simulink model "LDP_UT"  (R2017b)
settings: Solver=FixedStepDiscrete  StartTime=0.0  StopTime=10.0  FixedStep=0.01  RelTol=1e-3  EnableMultiTasking=on
undefined symbols (not defined in the file): ASWTYPE_FALSE, ASWTYPE_TRUE, CaCDP_ChrgTempNTCVoltTable_mV, CaCDP_ChrgTempTable_C, CaLDP_InletWtTempTable_C, CaLDP_InletWtVolt_mV, CaLDP_OutletWtTempTable_C, CaLDP_OutletWtVolt_mV, CcLDP_CC2SplyVolt_mV, CcLDP_CC2Uncon2ConTi_ms, CcLDP_CC2VoltThd_mV, CcLDP_DCChrgNegTempHiThrd_C, CcLDP_DCChrgNegTempMaxThrd_mV, CcLDP_DCChrgNegTempMinThrd_mV, CcLDP_DCChrgPosTempHiThrd_C, CcLDP_DCChrgPosTempMaxThrd_mV, CcLDP_DCChrgPosTempMinThrd_mV, CcLDP_DCSplyOnDebTi_ms, CcLDP_DCWakeVolt_V, CcLDP_IntWtTempHiThrd_C, CcLDP_IntWtTempMaxThrd_mV, CcLDP_IntWtTempMinThrd_mV, CcLDP_OutWtTempHiThrd_C, CcLDP_OutWtTempMaxThrd_mV, CcLDP_OutWtTempMinThrd_mV, Enum_CTCCtrCtlConnMode, Enum_LDPCC2St, Enum_LDPChrgGunState, Enum_ODPCCState, LDP_CONST2_NUMB, LDP_RUNTIME_MS
libraries: AIWAYS_Powertrain_BMS_lib x82
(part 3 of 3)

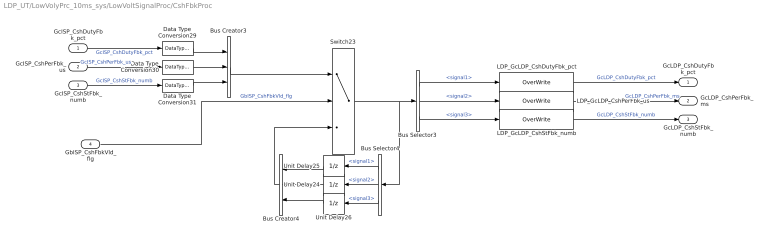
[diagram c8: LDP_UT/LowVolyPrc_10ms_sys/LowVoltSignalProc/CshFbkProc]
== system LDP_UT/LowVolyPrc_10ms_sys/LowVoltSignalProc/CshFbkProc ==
  GcISP_CshDutyFbk_pct : Inport
  GcISP_CshPerFbk_us : Inport  Port=2
  GcISP_CshStFbk_numb : Inport  Port=3
  GbISP_CshFbkVld_flg : Inport  Port=4
  Bus Creator3 : BusCreator  Inputs=3
  Bus Creator4 : BusCreator  Inputs=3
  Bus Selector3 : BusSelector  OutputSignals=signal1,signal2,signal3
  Bus Selector4 : BusSelector  OutputSignals=signal1,signal2,signal3
  Data Type Conversion29 : DataTypeConversion
  Data Type Conversion30 : DataTypeConversion
  Data Type Conversion31 : DataTypeConversion
  LDP_GcLDP_CshDutyFbk_pct : AIWAYS_Powertrain_BMS_lib/Signals/OverWrite  OverWrite_Value=CcLDP_CshDutyFbkOvr_pct  OverWrite_flag=CbLDP_CshDutyFbkOvrSwt_flg
  LDP_GcLDP_CshPerFbk_us : AIWAYS_Powertrain_BMS_lib/Signals/OverWrite  OverWrite_Value=CcLDP_CshPerFbkOvr_ms  OverWrite_flag=CbLDP_CshPerFbkOvrSwt_flg
  LDP_GcLDP_CshStFbk_numb : AIWAYS_Powertrain_BMS_lib/Signals/OverWrite  OverWrite_Value=CcLDP_CshStFbkOvr_numb  OverWrite_flag=CbLDP_CshStFbkOvrSwt_flg
  Switch23 : Switch  Criteria=u2 ~= 0  Threshold=1  RndMeth=Zero
  Unit Delay24 : UnitDelay  SampleTime=-1  StateName=StateName
  Unit Delay25 : UnitDelay  SampleTime=-1  StateName=StateName
  Unit Delay26 : UnitDelay  SampleTime=-1  StateName=StateName
  GcLDP_CshDutyFbk_pct : Outport
  GcLDP_CshPerFbk_ms : Outport  Port=2
  GcLDP_CshStFbk_numb : Outport  Port=3
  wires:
  Bus Selector4/2 -> Unit Delay24/1  "<signal2>"
  Bus Selector3/2 -> LDP_GcLDP_CshPerFbk_us/1  "<signal2>"
  LDP_GcLDP_CshDutyFbk_pct/1 -> GcLDP_CshDutyFbk_pct/1  "GcLDP_CshDutyFbk_pct"
  Bus Selector4/1 -> Unit Delay25/1  "<signal1>"
  Bus Selector3/1 -> LDP_GcLDP_CshDutyFbk_pct/1  "<signal1>"
  Unit Delay25/1 -> Bus Creator4/1
  Unit Delay26/1 -> Bus Creator4/3
  Unit Delay24/1 -> Bus Creator4/2
  GcISP_CshStFbk_numb/1 -> Data Type Conversion31/1  "GcISP_CshStFbk_numb"
  Bus Selector4/3 -> Unit Delay26/1  "<signal3>"
  GbISP_CshFbkVld_flg/1 -> Switch23/2  "GbISP_CshFbkVld_flg"
  Data Type Conversion31/1 -> Bus Creator3/3
  Data Type Conversion30/1 -> Bus Creator3/2
  Bus Creator3/1 -> Switch23/1
  Bus Selector3/3 -> LDP_GcLDP_CshStFbk_numb/1  "<signal3>"
  LDP_GcLDP_CshPerFbk_us/1 -> GcLDP_CshPerFbk_ms/1  "GcLDP_CshPerFbk_ms"
  Bus Creator4/1 -> Switch23/3
  GcISP_CshDutyFbk_pct/1 -> Data Type Conversion29/1  "GcISP_CshDutyFbk_pct"
  LDP_GcLDP_CshStFbk_numb/1 -> GcLDP_CshStFbk_numb/1  "GcLDP_CshStFbk_numb"
  Switch23/1 -> Bus Selector4/1, Bus Selector3/1
  GcISP_CshPerFbk_us/1 -> Data Type Conversion30/1  "GcISP_CshPerFbk_us"
  Data Type Conversion29/1 -> Bus Creator3/1

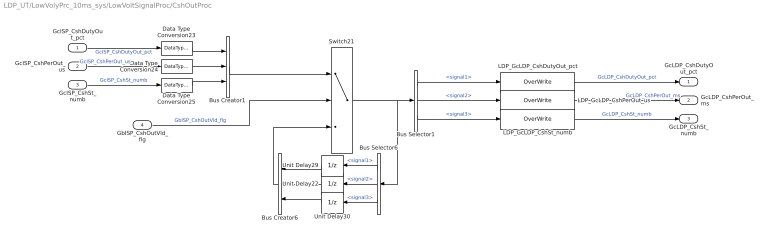
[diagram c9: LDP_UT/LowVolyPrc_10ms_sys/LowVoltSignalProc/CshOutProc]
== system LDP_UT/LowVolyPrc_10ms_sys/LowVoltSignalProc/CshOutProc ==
  GcISP_CshDutyOut_pct : Inport
  GcISP_CshPerOut_us : Inport  Port=2
  GcISP_CshSt_numb : Inport  Port=3
  GbISP_CshOutVld_flg : Inport  Port=4
  Bus Creator1 : BusCreator  Inputs=3
  Bus Creator6 : BusCreator  Inputs=3
  Bus Selector1 : BusSelector  OutputSignals=signal1,signal2,signal3
  Bus Selector6 : BusSelector  OutputSignals=signal1,signal2,signal3
  Data Type Conversion23 : DataTypeConversion
  Data Type Conversion24 : DataTypeConversion
  Data Type Conversion25 : DataTypeConversion
  LDP_GcLDP_CshDutyOut_pct : AIWAYS_Powertrain_BMS_lib/Signals/OverWrite  OverWrite_Value=CcLDP_CshDutyOutOvr_pct  OverWrite_flag=CbLDP_CshDutyOutOvrSwt_flg
  LDP_GcLDP_CshPerOut_us : AIWAYS_Powertrain_BMS_lib/Signals/OverWrite  OverWrite_Value=CcLDP_CshPerOutOvr_ms  OverWrite_flag=CbLDP_CshPerOutOvrSwt_flg
  LDP_GcLDP_CshSt_numb : AIWAYS_Powertrain_BMS_lib/Signals/OverWrite  OverWrite_Value=CcLDP_CshStOvr_numb  OverWrite_flag=CbLDP_CshStOvrSwt_flg
  Switch21 : Switch  Criteria=u2 ~= 0  Threshold=1  RndMeth=Zero
  Unit Delay22 : UnitDelay  SampleTime=-1  StateName=StateName
  Unit Delay29 : UnitDelay  SampleTime=-1  StateName=StateName
  Unit Delay30 : UnitDelay  SampleTime=-1  StateName=StateName
  GcLDP_CshDutyOut_pct : Outport
  GcLDP_CshPerOut_ms : Outport  Port=2
  GcLDP_CshSt_numb : Outport  Port=3
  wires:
  Data Type Conversion25/1 -> Bus Creator1/3
  Unit Delay22/1 -> Bus Creator6/2
  GcISP_CshSt_numb/1 -> Data Type Conversion25/1  "GcISP_CshSt_numb"
  Data Type Conversion23/1 -> Bus Creator1/1
  Bus Selector6/2 -> Unit Delay22/1  "<signal2>"
  Bus Creator6/1 -> Switch21/3
  Switch21/1 -> Bus Selector6/1, Bus Selector1/1
  LDP_GcLDP_CshDutyOut_pct/1 -> GcLDP_CshDutyOut_pct/1  "GcLDP_CshDutyOut_pct"
  Bus Selector6/1 -> Unit Delay29/1  "<signal1>"
  Unit Delay29/1 -> Bus Creator6/1
  Data Type Conversion24/1 -> Bus Creator1/2
  Bus Selector6/3 -> Unit Delay30/1  "<signal3>"
  Bus Selector1/2 -> LDP_GcLDP_CshPerOut_us/1  "<signal2>"
  GbISP_CshOutVld_flg/1 -> Switch21/2  "GbISP_CshOutVld_flg"
  Bus Selector1/1 -> LDP_GcLDP_CshDutyOut_pct/1  "<signal1>"
  Bus Selector1/3 -> LDP_GcLDP_CshSt_numb/1  "<signal3>"
  LDP_GcLDP_CshPerOut_us/1 -> GcLDP_CshPerOut_ms/1  "GcLDP_CshPerOut_ms"
  LDP_GcLDP_CshSt_numb/1 -> GcLDP_CshSt_numb/1  "GcLDP_CshSt_numb"
  Bus Creator1/1 -> Switch21/1
  GcISP_CshPerOut_us/1 -> Data Type Conversion24/1  "GcISP_CshPerOut_us"
  GcISP_CshDutyOut_pct/1 -> Data Type Conversion23/1  "GcISP_CshDutyOut_pct"
  Unit Delay30/1 -> Bus Creator6/3

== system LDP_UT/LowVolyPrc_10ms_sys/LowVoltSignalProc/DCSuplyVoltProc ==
  GcISP_DCSuplyVolt_mV : Inport
  GbISP_DCSuplyVoltVld_flg : Inport  Port=2
  Data Type Conversion1 : DataTypeConversion
  Data Type Conversion2 : DataTypeConversion
  Data Type Conversion4 : DataTypeConversion
  LDP_GbLDP_DCSuplyVoltVld_flg : AIWAYS_Powertrain_BMS_lib/Signals/OverWrite  OverWrite_Value=CbLDP_DCSuplyVoltVldOvr_flg  OverWrite_flag=CbLDP_DCSuplyVoltVldOvrSwt_flg
  LDP_GcLDP_DCSuplyVolt_mV : AIWAYS_Powertrain_BMS_lib/Signals/OverWrite  OverWrite_Value=CcLDP_DCSuplyVoltOvr_mV  OverWrite_flag=CbLDP_DCSuplyVoltOvrSwt_flg
  Switch4 : Switch  Criteria=u2 ~= 0
  Unit Delay4 : UnitDelay  SampleTime=-1  StateName=StateName
  GcLDP_DCSuplyVolt_mV : Outport
  GbLDP_DCSuplyVoltVld_flg : Outport  Port=2
  LbLDP_DCSuplyVoltVld_flg : Outport  Port=3
  LcLDP_DCSuplyVolt_mV : Outport  Port=4
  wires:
  Data Type Conversion4/1 -> Switch4/1
  Unit Delay4/1 -> Switch4/3
  Switch4/1 -> LDP_GcLDP_DCSuplyVolt_mV/1, Unit Delay4/1, Data Type Conversion2/1
  LDP_GcLDP_DCSuplyVolt_mV/1 -> GcLDP_DCSuplyVolt_mV/1  "GcLDP_DCSuplyVolt_mV"
  GbISP_DCSuplyVoltVld_flg/1 -> Data Type Conversion1/1, LDP_GbLDP_DCSuplyVoltVld_flg/1, Switch4/2  "GbISP_DCSuplyVoltVld_flg"
  GcISP_DCSuplyVolt_mV/1 -> Data Type Conversion4/1  "GcISP_DCSuplyVolt_mV"
  LDP_GbLDP_DCSuplyVoltVld_flg/1 -> GbLDP_DCSuplyVoltVld_flg/1  "GbLDP_DCSuplyVoltVld_flg"
  Data Type Conversion1/1 -> LbLDP_DCSuplyVoltVld_flg/1  "LbLDP_DCSuplyVoltVld_flg"
  Data Type Conversion2/1 -> LcLDP_DCSuplyVolt_mV/1  "LcLDP_DCSuplyVolt_mV"

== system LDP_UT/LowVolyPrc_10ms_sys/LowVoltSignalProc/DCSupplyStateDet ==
  LbLDP_DCSuplyVoltVld_flg : Inport
  LcLDP_DCSuplyVolt_mV : Inport  Port=2
  BMSDebounceStartZero1 : AIWAYS_Powertrain_BMS_lib/Debounce & Delay/BMSDebounceStartZero
  Constant1 : Constant  Value=ASWTYPE_TRUE
  KeMDPR_t_EngChrgBatIdleMinSetTm10 : Constant  Value=CcLDP_DCSplyOnDebTi_ms
  KeMDPR_t_EngChrgBatIdleMinSetTm2 : Constant  Value=LDP_RUNTIME_MS
  KeMDPR_t_EngChrgBatIdleMinSetTm3 : Constant  Value=LDP_RUNTIME_MS
  KeMDPR_t_EngChrgBatIdleMinSetTm6 : Constant  Value=CcLDP_DCWakeVolt_V
  KeMDPR_t_EngChrgBatIdleMinSetTm9 : Constant  Value=CcLDP_DCSplyOnDebTi_ms
  LDP_GbLDP_DC12VSply_flg : AIWAYS_Powertrain_BMS_lib/Signals/OverWrite  OverWrite_Value=CbLDP_DC12VSplyOvr_flg  OverWrite_flag=CbLDP_DC12VSplyOvrSwt_flg
  Logical Operator2 : Logic  AllPortsSameDT=off  OutDataTypeStr=boolean
  Relational Operator3 : RelationalOperator  OutDataTypeStr=boolean
  Relational Operator4 : RelationalOperator  Operator===  OutDataTypeStr=boolean
  GbLDP_DC12VSply_flg : Outport
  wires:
  LDP_GbLDP_DC12VSply_flg/1 -> GbLDP_DC12VSply_flg/1  "GbLDP_DC12VSply_flg"
  LcLDP_DCSuplyVolt_mV/1 -> Relational Operator3/1
  LbLDP_DCSuplyVoltVld_flg/1 -> Relational Operator4/1
  Constant1/1 -> Relational Operator4/2
  Relational Operator3/1 -> Logical Operator2/1
  Relational Operator4/1 -> Logical Operator2/2
  Logical Operator2/1 -> BMSDebounceStartZero1/1
  BMSDebounceStartZero1/1 -> LDP_GbLDP_DC12VSply_flg/1
  KeMDPR_t_EngChrgBatIdleMinSetTm2/1 -> BMSDebounceStartZero1/3
  KeMDPR_t_EngChrgBatIdleMinSetTm3/1 -> BMSDebounceStartZero1/5
  KeMDPR_t_EngChrgBatIdleMinSetTm6/1 -> Relational Operator3/2
  KeMDPR_t_EngChrgBatIdleMinSetTm9/1 -> BMSDebounceStartZero1/2
  KeMDPR_t_EngChrgBatIdleMinSetTm10/1 -> BMSDebounceStartZero1/4

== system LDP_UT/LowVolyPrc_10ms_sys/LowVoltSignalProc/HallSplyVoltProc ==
  GbISP_HallSplyVoltVld_flg : Inport
  GcISP_HallSplyVolt_mV : Inport  Port=2
  Data Type Conversion2 : DataTypeConversion
  LDP_GbLDP_HallSplyVoltVld_flg : AIWAYS_Powertrain_BMS_lib/Signals/OverWrite  OverWrite_Value=CbLDP_HallSplyVoltVldOvr_flg  OverWrite_flag=CbLDP_HallSplyVoltVldOvrSwt_flg
  LDP_GcLDP_HallSplyVolt_mV : AIWAYS_Powertrain_BMS_lib/Signals/OverWrite  OverWrite_Value=CcLDP_HallSplyVoltOvr_mV  OverWrite_flag=CbLDP_HallSplyVoltOvrSwt_flg
  Switch2 : Switch  Criteria=u2 ~= 0
  Unit Delay2 : UnitDelay  SampleTime=-1  StateName=StateName
  GcLDP_HallSplyVolt_mV : Outport
  GbLDP_HallSplyVoltVld_flg : Outport  Port=2
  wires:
  Data Type Conversion2/1 -> Switch2/1
  Unit Delay2/1 -> Switch2/3
  GbISP_HallSplyVoltVld_flg/1 -> LDP_GbLDP_HallSplyVoltVld_flg/1, Switch2/2  "GbISP_HallSplyVoltVld_flg"
  LDP_GbLDP_HallSplyVoltVld_flg/1 -> GbLDP_HallSplyVoltVld_flg/1  "GbLDP_HallSplyVoltVld_flg"
  GcISP_HallSplyVolt_mV/1 -> Data Type Conversion2/1  "GcISP_HallSplyVolt_mV"
  Switch2/1 -> Unit Delay2/1, LDP_GcLDP_HallSplyVolt_mV/1
  LDP_GcLDP_HallSplyVolt_mV/1 -> GcLDP_HallSplyVolt_mV/1  "GcLDP_HallSplyVolt_mV"

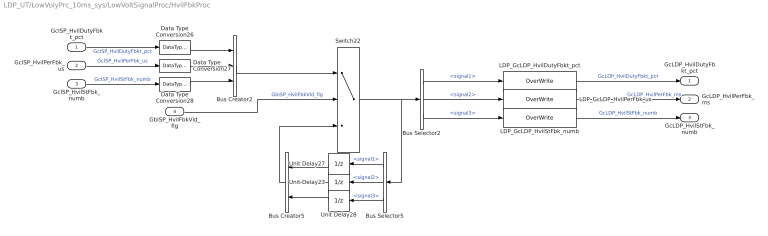
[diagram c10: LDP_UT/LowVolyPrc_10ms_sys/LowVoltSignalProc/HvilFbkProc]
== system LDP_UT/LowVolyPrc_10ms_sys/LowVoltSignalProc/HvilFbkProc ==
  GcISP_HvilDutyFbkt_pct : Inport
  GcISP_HvilPerFbk_us : Inport  Port=2
  GcISP_HvilStFbk_numb : Inport  Port=3
  GbISP_HvilFbkVld_flg : Inport  Port=4
  Bus Creator2 : BusCreator  Inputs=3
  Bus Creator5 : BusCreator  Inputs=3
  Bus Selector2 : BusSelector  OutputSignals=signal1,signal2,signal3
  Bus Selector5 : BusSelector  OutputSignals=signal1,signal2,signal3
  Data Type Conversion26 : DataTypeConversion
  Data Type Conversion27 : DataTypeConversion
  Data Type Conversion28 : DataTypeConversion
  LDP_GcLDP_HvilDutyFbkt_pct : AIWAYS_Powertrain_BMS_lib/Signals/OverWrite  OverWrite_Value=CcLDP_HvilDutyFbktOvr_pct  OverWrite_flag=CbLDP_HvilDutyFbktOvrSwt_flg
  LDP_GcLDP_HvilPerFbk_us : AIWAYS_Powertrain_BMS_lib/Signals/OverWrite  OverWrite_Value=CcLDP_HvilPerFbkOvr_ms  OverWrite_flag=CbLDP_HvilPerFbkOvrSwt_flg
  LDP_GcLDP_HvilStFbk_numb : AIWAYS_Powertrain_BMS_lib/Signals/OverWrite  OverWrite_Value=CcLDP_HvilStFbkOvr_numb  OverWrite_flag=CbLDP_HvilStFbkOvrSwt_flg
  Switch22 : Switch  Criteria=u2 ~= 0  Threshold=1  RndMeth=Zero
  Unit Delay23 : UnitDelay  SampleTime=-1  StateName=StateName
  Unit Delay27 : UnitDelay  SampleTime=-1  StateName=StateName
  Unit Delay28 : UnitDelay  SampleTime=-1  StateName=StateName
  GcLDP_HvilDutyFbkt_pct : Outport
  GcLDP_HvilPerFbk_ms : Outport  Port=2
  GcLDP_HvilStFbk_numb : Outport  Port=3
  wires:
  Switch22/1 -> Bus Selector5/1, Bus Selector2/1
  Data Type Conversion26/1 -> Bus Creator2/1
  Unit Delay23/1 -> Bus Creator5/2
  LDP_GcLDP_HvilStFbk_numb/1 -> GcLDP_HvilStFbk_numb/1  "GcLDP_HvilStFbk_numb"
  Bus Selector5/3 -> Unit Delay28/1  "<signal3>"
  Bus Selector5/2 -> Unit Delay23/1  "<signal2>"
  Bus Selector5/1 -> Unit Delay27/1  "<signal1>"
  Bus Creator5/1 -> Switch22/3
  Bus Selector2/2 -> LDP_GcLDP_HvilPerFbk_us/1  "<signal2>"
  Unit Delay28/1 -> Bus Creator5/3
  Unit Delay27/1 -> Bus Creator5/1
  GcISP_HvilDutyFbkt_pct/1 -> Data Type Conversion26/1  "GcISP_HvilDutyFbkt_pct"
  Data Type Conversion28/1 -> Bus Creator2/3
  Bus Creator2/1 -> Switch22/1
  Data Type Conversion27/1 -> Bus Creator2/2
  GcISP_HvilPerFbk_us/1 -> Data Type Conversion27/1  "GcISP_HvilPerFbk_us"
  LDP_GcLDP_HvilPerFbk_us/1 -> GcLDP_HvilPerFbk_ms/1  "GcLDP_HvilPerFbk_ms"
  LDP_GcLDP_HvilDutyFbkt_pct/1 -> GcLDP_HvilDutyFbkt_pct/1  "GcLDP_HvilDutyFbkt_pct"
  Bus Selector2/3 -> LDP_GcLDP_HvilStFbk_numb/1  "<signal3>"
  GcISP_HvilStFbk_numb/1 -> Data Type Conversion28/1  "GcISP_HvilStFbk_numb"
  Bus Selector2/1 -> LDP_GcLDP_HvilDutyFbkt_pct/1  "<signal1>"
  GbISP_HvilFbkVld_flg/1 -> Switch22/2  "GbISP_HvilFbkVld_flg"

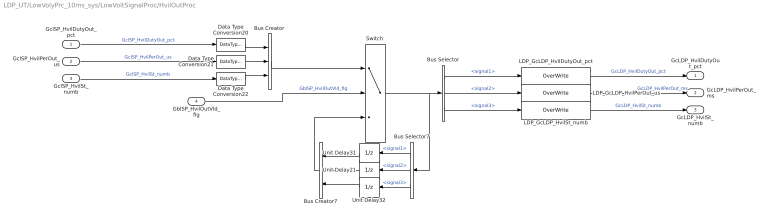
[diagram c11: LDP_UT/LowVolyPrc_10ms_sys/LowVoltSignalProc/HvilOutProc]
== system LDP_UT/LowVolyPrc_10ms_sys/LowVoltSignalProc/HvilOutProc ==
  GcISP_HvilDutyOut_pct : Inport
  GcISP_HvilPerOut_us : Inport  Port=2
  GcISP_HvilSt_numb : Inport  Port=3
  GbISP_HvilOutVld_flg : Inport  Port=4
  Bus Creator : BusCreator  Inputs=3
  Bus Creator7 : BusCreator  Inputs=3
  Bus Selector : BusSelector  OutputSignals=signal1,signal2,signal3
  Bus Selector7 : BusSelector  OutputSignals=signal1,signal2,signal3
  Data Type Conversion20 : DataTypeConversion
  Data Type Conversion21 : DataTypeConversion
  Data Type Conversion22 : DataTypeConversion
  LDP_GcLDP_HvilDutyOut_pct : AIWAYS_Powertrain_BMS_lib/Signals/OverWrite  OverWrite_Value=CcLDP_HvilDutyOutOvr_pct  OverWrite_flag=CbLDP_HvilDutyOutOvrSwt_flg
  LDP_GcLDP_HvilPerOut_us : AIWAYS_Powertrain_BMS_lib/Signals/OverWrite  OverWrite_Value=CcLDP_HvilPerOutOvr_ms  OverWrite_flag=CbLDP_HvilPerOutOvrSwt_flg
  LDP_GcLDP_HvilSt_numb : AIWAYS_Powertrain_BMS_lib/Signals/OverWrite  OverWrite_Value=CcLDP_HvilStOvr_numb  OverWrite_flag=CbLDP_HvilStOvrSwt_flg
  Switch : Switch  Criteria=u2 ~= 0  Threshold=1  RndMeth=Zero
  Unit Delay21 : UnitDelay  SampleTime=-1  StateName=StateName
  Unit Delay31 : UnitDelay  SampleTime=-1  StateName=StateName
  Unit Delay32 : UnitDelay  SampleTime=-1  StateName=StateName
  GcLDP_HvilDutyOut_pct : Outport
  GcLDP_HvilPerOut_ms : Outport  Port=2
  GcLDP_HvilSt_numb : Outport  Port=3
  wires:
  Bus Selector/1 -> LDP_GcLDP_HvilDutyOut_pct/1  "<signal1>"
  Bus Selector7/2 -> Unit Delay21/1  "<signal2>"
  Unit Delay32/1 -> Bus Creator7/3
  Bus Selector7/1 -> Unit Delay31/1  "<signal1>"
  Bus Creator7/1 -> Switch/3
  GcISP_HvilDutyOut_pct/1 -> Data Type Conversion20/1  "GcISP_HvilDutyOut_pct"
  Unit Delay21/1 -> Bus Creator7/2
  Unit Delay31/1 -> Bus Creator7/1
  GbISP_HvilOutVld_flg/1 -> Switch/2  "GbISP_HvilOutVld_flg"
  GcISP_HvilSt_numb/1 -> Data Type Conversion22/1  "GcISP_HvilSt_numb"
  Data Type Conversion22/1 -> Bus Creator/3
  Switch/1 -> Bus Selector7/1, Bus Selector/1
  Bus Selector/3 -> LDP_GcLDP_HvilSt_numb/1  "<signal3>"
  Bus Creator/1 -> Switch/1
  LDP_GcLDP_HvilPerOut_us/1 -> GcLDP_HvilPerOut_ms/1  "GcLDP_HvilPerOut_ms"
  Bus Selector7/3 -> Unit Delay32/1  "<signal3>"
  Data Type Conversion20/1 -> Bus Creator/1
  Bus Selector/2 -> LDP_GcLDP_HvilPerOut_us/1  "<signal2>"
  LDP_GcLDP_HvilSt_numb/1 -> GcLDP_HvilSt_numb/1  "GcLDP_HvilSt_numb"
  LDP_GcLDP_HvilDutyOut_pct/1 -> GcLDP_HvilDutyOut_pct/1  "GcLDP_HvilDutyOut_pct"
  GcISP_HvilPerOut_us/1 -> Data Type Conversion21/1  "GcISP_HvilPerOut_us"
  Data Type Conversion21/1 -> Bus Creator/2

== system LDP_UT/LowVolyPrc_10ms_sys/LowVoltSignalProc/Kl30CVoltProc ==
  GcISP_Kl30CVolt_mV : Inport
  GbISP_Kl30CVoltVld_flg : Inport  Port=2
  Data Type Conversion5 : DataTypeConversion
  LDP_GbLDP_Kl30CVoltVld_flg : AIWAYS_Powertrain_BMS_lib/Signals/OverWrite  OverWrite_Value=CbLDP_Kl30CVoltVldOvr_flg  OverWrite_flag=CbLDP_Kl30CVoltVldOvrSwt_flg
  LDP_GcLDP_Kl30CVolt_mV : AIWAYS_Powertrain_BMS_lib/Signals/OverWrite  OverWrite_Value=CcLDP_Kl30CVoltOvr_mV  OverWrite_flag=CbLDP_Kl30CVoltOvrSwt_flg
  Switch5 : Switch  Criteria=u2 ~= 0
  Unit Delay5 : UnitDelay  SampleTime=-1  StateName=StateName
  GcLDP_Kl30CVolt_mV : Outport
  GbLDP_Kl30CVoltVld_flg : Outport  Port=2
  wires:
  GcISP_Kl30CVolt_mV/1 -> Data Type Conversion5/1  "GcISP_Kl30CVolt_mV"
  Switch5/1 -> LDP_GcLDP_Kl30CVolt_mV/1, Unit Delay5/1
  Unit Delay5/1 -> Switch5/3
  GbISP_Kl30CVoltVld_flg/1 -> Switch5/2, LDP_GbLDP_Kl30CVoltVld_flg/1  "GbISP_Kl30CVoltVld_flg"
  LDP_GcLDP_Kl30CVolt_mV/1 -> GcLDP_Kl30CVolt_mV/1  "GcLDP_Kl30CVolt_mV"
  LDP_GbLDP_Kl30CVoltVld_flg/1 -> GbLDP_Kl30CVoltVld_flg/1  "GbLDP_Kl30CVoltVld_flg"
  Data Type Conversion5/1 -> Switch5/1

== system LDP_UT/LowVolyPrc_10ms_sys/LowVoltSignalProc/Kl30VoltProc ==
  GbISP_Kl30VoltVld_flg : Inport
  GcISP_Kl30Volt_mV : Inport  Port=2
  Data Type Conversion6 : DataTypeConversion
  LDP_GbLDP_Kl30VoltVld_flg : AIWAYS_Powertrain_BMS_lib/Signals/OverWrite  OverWrite_Value=CbLDP_Kl30VoltVldOvr_flg  OverWrite_flag=CbLDP_Kl30VoltVldOvrSwt_flg
  LDP_GcLDP_Kl30Volt_mV : AIWAYS_Powertrain_BMS_lib/Signals/OverWrite  OverWrite_Value=CcLDP_Kl30VoltOvr_mV  OverWrite_flag=CbLDP_Kl30VoltOvrSwt_flg
  Switch6 : Switch  Criteria=u2 ~= 0
  Unit Delay6 : UnitDelay  SampleTime=-1  StateName=StateName
  GcLDP_Kl30Volt_mV : Outport
  GbLDP_Kl30VoltVld_flg : Outport  Port=2
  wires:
  LDP_GbLDP_Kl30VoltVld_flg/1 -> GbLDP_Kl30VoltVld_flg/1  "GbLDP_Kl30VoltVld_flg"
  GbISP_Kl30VoltVld_flg/1 -> LDP_GbLDP_Kl30VoltVld_flg/1, Switch6/2  "GbISP_Kl30VoltVld_flg"
  Unit Delay6/1 -> Switch6/3
  LDP_GcLDP_Kl30Volt_mV/1 -> GcLDP_Kl30Volt_mV/1  "GcLDP_Kl30Volt_mV"
  GcISP_Kl30Volt_mV/1 -> Data Type Conversion6/1  "GcISP_Kl30Volt_mV"
  Switch6/1 -> LDP_GcLDP_Kl30Volt_mV/1, Unit Delay6/1
  Data Type Conversion6/1 -> Switch6/1

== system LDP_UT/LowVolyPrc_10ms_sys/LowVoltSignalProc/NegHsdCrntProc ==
  GcISP_NegHsdCrnt_mV : Inport
  GbISP_NegHsdCrntVld_flg : Inport  Port=2
  Data Type Conversion9 : DataTypeConversion
  LDP_GbLDP_NegHsdCrntVld_flg : AIWAYS_Powertrain_BMS_lib/Signals/OverWrite  OverWrite_Value=CbLDP_NegHsdCrntVldOvr_flg  OverWrite_flag=CbLDP_NegHsdCrntVldOvrSwt_flg
  LDP_GcLDP_NegHsdCrnt_mV : AIWAYS_Powertrain_BMS_lib/Signals/OverWrite  OverWrite_Value=CcLDP_NegHsdCrntOvr_mV  OverWrite_flag=CbLDP_NegHsdCrntOvrSwt_flg
  Switch9 : Switch  Criteria=u2 ~= 0
  Unit Delay9 : UnitDelay  SampleTime=-1  StateName=StateName
  GcLDP_NegHsdCrnt_mV : Outport
  GbLDP_NegHsdCrntVld_flg : Outport  Port=2
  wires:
  Switch9/1 -> LDP_GcLDP_NegHsdCrnt_mV/1, Unit Delay9/1
  LDP_GbLDP_NegHsdCrntVld_flg/1 -> GbLDP_NegHsdCrntVld_flg/1  "GbLDP_NegHsdCrntVld_flg"
  Unit Delay9/1 -> Switch9/3
  LDP_GcLDP_NegHsdCrnt_mV/1 -> GcLDP_NegHsdCrnt_mV/1  "GcLDP_NegHsdCrnt_mV"
  GcISP_NegHsdCrnt_mV/1 -> Data Type Conversion9/1  "GcISP_NegHsdCrnt_mV"
  GbISP_NegHsdCrntVld_flg/1 -> LDP_GbLDP_NegHsdCrntVld_flg/1, Switch9/2  "GbISP_NegHsdCrntVld_flg"
  Data Type Conversion9/1 -> Switch9/1

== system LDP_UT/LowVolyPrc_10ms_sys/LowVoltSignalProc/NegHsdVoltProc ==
  GcISP_NegHsdVolt_mV : Inport
  GbISP_NegHsdVoltVld_flg : Inport  Port=2
  Data Type Conversion11 : DataTypeConversion
  LDP_GbLDP_NegHsdVoltVld_flg : AIWAYS_Powertrain_BMS_lib/Signals/OverWrite  OverWrite_Value=CbLDP_NegHsdVoltVldOvr_flg  OverWrite_flag=CbLDP_NegHsdVoltVldOvrSwt_flg
  LDP_GcLDP_NegHsdVolt_mV : AIWAYS_Powertrain_BMS_lib/Signals/OverWrite  OverWrite_Value=CcLDP_NegHsdVoltOvr_mV  OverWrite_flag=CbLDP_NegHsdVoltOvrSwt_flg
  Switch11 : Switch  Criteria=u2 ~= 0
  Unit Delay11 : UnitDelay  SampleTime=-1  StateName=StateName
  GcLDP_NegHsdVolt_mV : Outport
  GbLDP_NegHsdVoltVld_flg : Outport  Port=2
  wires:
  LDP_GbLDP_NegHsdVoltVld_flg/1 -> GbLDP_NegHsdVoltVld_flg/1  "GbLDP_NegHsdVoltVld_flg"
  Unit Delay11/1 -> Switch11/3
  Data Type Conversion11/1 -> Switch11/1
  GbISP_NegHsdVoltVld_flg/1 -> LDP_GbLDP_NegHsdVoltVld_flg/1, Switch11/2  "GbISP_NegHsdVoltVld_flg"
  Switch11/1 -> LDP_GcLDP_NegHsdVolt_mV/1, Unit Delay11/1
  LDP_GcLDP_NegHsdVolt_mV/1 -> GcLDP_NegHsdVolt_mV/1  "GcLDP_NegHsdVolt_mV"
  GcISP_NegHsdVolt_mV/1 -> Data Type Conversion11/1  "GcISP_NegHsdVolt_mV"

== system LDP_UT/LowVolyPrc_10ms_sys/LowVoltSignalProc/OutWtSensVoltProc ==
  GcISP_OutWtSensVolt_mV : Inport
  GbISP_OutWtSensVoltVld_flg : Inport  Port=2
  1-D Lookup Table3 : Lookup_n-D  NumberOfTableDimensions=1  BreakpointsForDimension1=CaLDP_OutletWtVolt_mV  Table=CaLDP_OutletWtTempTable_C  ExtrapMethod=Clip  UseLastTableValue=on  InternalRulePriority=Speed  OutDataTypeStr=Inherit: Inherit from 'Table data'  RndMeth=Simplest
  Data Type Conversion17 : DataTypeConversion
  LDP_GbLDP_OutWtSensVoltVld_flg : AIWAYS_Powertrain_BMS_lib/Signals/OverWrite  OverWrite_Value=CbLDP_OutWtSensVoltVldOvr_flg  OverWrite_flag=CbLDP_OutWtSensVoltVldOvrSwt_flg
  LDP_GcLDP_OutWtTemp_C : AIWAYS_Powertrain_BMS_lib/Signals/OverWrite  OverWrite_Value=CcLDP_OutWtTempOvr_C  OverWrite_flag=CbLDP_OutWtTempOvrSwt_flg
  Switch17 : Switch  Criteria=u2 ~= 0
  Unit Delay17 : UnitDelay  SampleTime=-1  StateName=StateName
  GbLDP_OutWtSensVoltVld_flg : Outport
  GcLDP_OutWtTemp_C : Outport  Port=2
  LcLDP_OutWtSensVolt_mV : Outport  Port=3
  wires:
  Data Type Conversion17/1 -> Switch17/1
  GbISP_OutWtSensVoltVld_flg/1 -> LDP_GbLDP_OutWtSensVoltVld_flg/1, Switch17/2  "GbISP_OutWtSensVoltVld_flg"
  LDP_GbLDP_OutWtSensVoltVld_flg/1 -> GbLDP_OutWtSensVoltVld_flg/1  "GbLDP_OutWtSensVoltVld_flg"
  Unit Delay17/1 -> Switch17/3
  GcISP_OutWtSensVolt_mV/1 -> Data Type Conversion17/1  "GcISP_OutWtSensVolt_mV"
  Switch17/1 -> 1-D Lookup Table3/1, LcLDP_OutWtSensVolt_mV/1, Unit Delay17/1  "LcLDP_OutWtSensVolt_mV"
  LDP_GcLDP_OutWtTemp_C/1 -> GcLDP_OutWtTemp_C/1  "GcLDP_OutWtTemp_C"
  1-D Lookup Table3/1 -> LDP_GcLDP_OutWtTemp_C/1

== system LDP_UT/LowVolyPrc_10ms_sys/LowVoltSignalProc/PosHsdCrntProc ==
  GcISP_PosHsdCrnt_mV : Inport
  GbISP_PosHsdCrntVld_flg : Inport  Port=2
  Data Type Conversion7 : DataTypeConversion
  LDP_GbLDP_PosHsdCrntVld_flg : AIWAYS_Powertrain_BMS_lib/Signals/OverWrite  OverWrite_Value=CbLDP_PosHsdCrntVldOvr_flg  OverWrite_flag=CbLDP_PosHsdCrntVldOvrSwt_flg
  LDP_GcLDP_PosHsdCrnt_mV : AIWAYS_Powertrain_BMS_lib/Signals/OverWrite  OverWrite_Value=CcLDP_PosHsdCrntOvr_mV  OverWrite_flag=CbLDP_PosHsdCrntOvrSwt_flg
  Switch7 : Switch  Criteria=u2 ~= 0
  Unit Delay7 : UnitDelay  SampleTime=-1  StateName=StateName
  GcLDP_PosHsdCrnt_mV : Outport
  GbLDP_PosHsdCrntVld_flg : Outport  Port=2
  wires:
  Switch7/1 -> LDP_GcLDP_PosHsdCrnt_mV/1, Unit Delay7/1
  GbISP_PosHsdCrntVld_flg/1 -> LDP_GbLDP_PosHsdCrntVld_flg/1, Switch7/2  "GbISP_PosHsdCrntVld_flg"
  GcISP_PosHsdCrnt_mV/1 -> Data Type Conversion7/1  "GcISP_PosHsdCrnt_mV"
  LDP_GbLDP_PosHsdCrntVld_flg/1 -> GbLDP_PosHsdCrntVld_flg/1  "GbLDP_PosHsdCrntVld_flg"
  LDP_GcLDP_PosHsdCrnt_mV/1 -> GcLDP_PosHsdCrnt_mV/1  "GcLDP_PosHsdCrnt_mV"
  Data Type Conversion7/1 -> Switch7/1
  Unit Delay7/1 -> Switch7/3

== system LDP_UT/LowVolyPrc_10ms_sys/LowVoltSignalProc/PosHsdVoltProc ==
  GcISP_PosHsdVolt_mV : Inport
  GbISP_PosHsdVoltVld_flg : Inport  Port=2
  Data Type Conversion10 : DataTypeConversion
  LDP_GbLDP_PosHsdVoltVld_flg : AIWAYS_Powertrain_BMS_lib/Signals/OverWrite  OverWrite_Value=CbLDP_PosHsdVoltVldOvr_flg  OverWrite_flag=CbLDP_PosHsdVoltVldOvrSwt_flg
  LDP_GcLDP_PosHsdVolt_mV : AIWAYS_Powertrain_BMS_lib/Signals/OverWrite  OverWrite_Value=CcLDP_PosHsdVoltOvr_mV  OverWrite_flag=CbLDP_PosHsdVoltOvrSwt_flg
  Switch10 : Switch  Criteria=u2 ~= 0
  Unit Delay10 : UnitDelay  SampleTime=-1  StateName=StateName
  GcLDP_PosHsdVolt_mV : Outport
  GbLDP_PosHsdVoltVld_flg : Outport  Port=2
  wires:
  LDP_GbLDP_PosHsdVoltVld_flg/1 -> GbLDP_PosHsdVoltVld_flg/1  "GbLDP_PosHsdVoltVld_flg"
  GcISP_PosHsdVolt_mV/1 -> Data Type Conversion10/1  "GcISP_PosHsdVolt_mV"
  Data Type Conversion10/1 -> Switch10/1
  Unit Delay10/1 -> Switch10/3
  GbISP_PosHsdVoltVld_flg/1 -> LDP_GbLDP_PosHsdVoltVld_flg/1, Switch10/2  "GbISP_PosHsdVoltVld_flg"
  LDP_GcLDP_PosHsdVolt_mV/1 -> GcLDP_PosHsdVolt_mV/1  "GcLDP_PosHsdVolt_mV"
  Switch10/1 -> LDP_GcLDP_PosHsdVolt_mV/1, Unit Delay10/1

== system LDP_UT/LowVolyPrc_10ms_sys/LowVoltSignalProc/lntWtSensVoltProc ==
  GcISP_lntWtSensVolt_mV : Inport
  GbISP_lntWtSensVoltVld_flg : Inport  Port=2
  1-D Lookup Table2 : Lookup_n-D  NumberOfTableDimensions=1  BreakpointsForDimension1=CaLDP_InletWtVolt_mV  Table=CaLDP_InletWtTempTable_C  ExtrapMethod=Clip  UseLastTableValue=on  InternalRulePriority=Speed  OutDataTypeStr=Inherit: Inherit from 'Table data'  RndMeth=Simplest
  Data Type Conversion16 : DataTypeConversion
  LDP_GbLDP_lntWtSensVoltVld_flg : AIWAYS_Powertrain_BMS_lib/Signals/OverWrite  OverWrite_Value=CbLDP_lntWtSensVoltVldOvr_flg  OverWrite_flag=CbLDP_lntWtSensVoltVldOvrSwt_flg
  LDP_GcLDP_lntWtTemp_C : AIWAYS_Powertrain_BMS_lib/Signals/OverWrite  OverWrite_Value=CcLDP_lntWtTempOvr_C  OverWrite_flag=CbLDP_lntWtTempOvrSwt_flg
  Switch16 : Switch  Criteria=u2 ~= 0
  Unit Delay16 : UnitDelay  SampleTime=-1  StateName=StateName
  GbLDP_lntWtSensVoltVld_flg : Outport
  GcLDP_lntWtTemp_C : Outport  Port=2
  LcLDP_lntWtSensVolt_mV : Outport  Port=3
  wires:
  LDP_GbLDP_lntWtSensVoltVld_flg/1 -> GbLDP_lntWtSensVoltVld_flg/1  "GbLDP_lntWtSensVoltVld_flg"
  Data Type Conversion16/1 -> Switch16/1
  Switch16/1 -> Unit Delay16/1, LcLDP_lntWtSensVolt_mV/1, 1-D Lookup Table2/1  "LcLDP_lntWtSensVolt_mV"
  GbISP_lntWtSensVoltVld_flg/1 -> LDP_GbLDP_lntWtSensVoltVld_flg/1, Switch16/2  "GbISP_lntWtSensVoltVld_flg"
  Unit Delay16/1 -> Switch16/3
  GcISP_lntWtSensVolt_mV/1 -> Data Type Conversion16/1  "GcISP_lntWtSensVolt_mV"
  1-D Lookup Table2/1 -> LDP_GcLDP_lntWtTemp_C/1
  LDP_GcLDP_lntWtTemp_C/1 -> GcLDP_lntWtTemp_C/1  "GcLDP_lntWtTemp_C"
